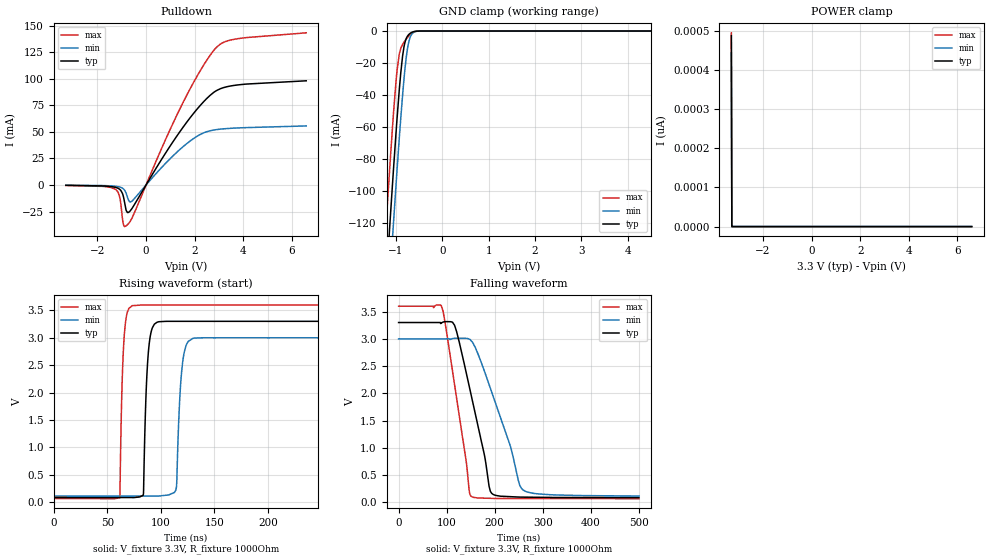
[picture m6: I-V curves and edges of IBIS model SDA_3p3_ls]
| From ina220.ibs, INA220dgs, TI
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|   Model
[Model]   SDA_3p3_ls
Model_type   I/O_open_drain
Polarity   Non-Inverting
Enable   Active-Low
Vinl = 0.99
Vinh = 2.31
Vmeas = 1.65
Vref = 3.3
Cref = 1pF
Rref = 1000
|   typ   min   max
C_comp   2.2433820E-12   1.9359850E-12 2.5433970E-12
[Voltage Range]   3.3   3   3.6
[Temperature Range]   27   85   -40
[Pullup Reference]   3.3   3   3.6
[Pulldown Reference]   -0   -0   -0
[Power Clamp Reference]   3.3   3   3.6
[GND Clamp Reference]   -0   -0   -0
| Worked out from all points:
|   slope of the pulldown table from 0 to 0.495 V, typ, clamps not added: 26.3 ohm
|   GND clamp passes 1 mA (typ) near -0.67 V on its own axis
|   falling waveform, V_fixture 3.3V, R_fixture 1000Ohm: 20-80 % time 47.7ns typ, 63.9ns min, 36.4ns max; typ from 3.3 V to 0.084 V
|   rising waveform, V_fixture 3.3V, R_fixture 1000Ohm: 20-80 % time 3.64ns typ, 4.29ns min, 3.07ns max; typ from 0.083 V to 3.3 V
[Pulldown]
|   Voltage   I(typ)   I(min)   I(max)
-3.3V     -316.9uA   -207.5uA   -421.7uA
-1.261V   -2.207mA   -1.204mA   -4.07mA
-1.102V   -3.787mA   -1.819mA   -9.812mA
-973.5mV  -7.834mA   -2.97mA    -31.07mA
-914.1mV  -12.66mA   -4.043mA   -38.45mA
-825mV    -23.31mA   -7.395mA   -38.56mA
-696.3mV  -25.37mA   -15.33mA   -35.64mA
-587.4mV  -22.38mA   -15.34mA   -31.61mA
1.393V    50.19mA    33.45mA    71.66mA
2.848V    88.14mA    51.95mA    128.4mA
3.61V     93.69mA    53.51mA    137.1mA
6.59V     98.08mA    55.58mA    143.2mA
[GND Clamp]
|   Voltage   I(typ)   I(min)   I(max)
-3.3V     -1.176A    -1.208A    -1.142A
-1.221V   -162.6mA   -196.9mA   -125.6mA
-1.132V   -122mA     -156mA     -85.52mA
-1.073V   -95.72mA   -129.4mA   -60.19mA
-1.053V   -87.15mA   -120.6mA   -52.17mA
-973.5mV  -54.4mA    -86.43mA   -24.47mA
-924mV    -35.97mA   -66.11mA   -14.02mA
-854.7mV  -15.61mA   -39.98mA   -8.368mA
-805.2mV  -7.274mA   -24.13mA   -6.138mA
-755.7mV  -3.503mA   -12.19mA   -4.229mA
-646.8mV  -706.8uA   -1.595mA   -1.161mA
6.59V     0A         0A         0A
[POWER Clamp]
|   Voltage   I(typ)   I(min)   I(max)
-3.3V     487.8pA    443.7pA    495.1pA
-3.28V    0A         0A         0A
-3.27V    0A         0A         0A
6.59V     0A         0A         0A
[Ramp]
R_load = 1000
|   typ   min   max
dV/dt_r   1.93018/3.63153e-09   1.73473/4.27814e-09   2.12159/3.0581e-09
dV/dt_f   1.92984/4.7651e-08   1.73215/6.39826e-08   2.12156/3.64371e-08
[Falling Waveform]
V_fixture = 3.3V
V_fixture_min = 3V
V_fixture_max = 3.6V
R_fixture = 1000Ohm
C_fixture = 0F
|   Time   V(typ)   V(min)   V(max)
0s        3.3V       3V         3.6V
88.8ns    3.289V     3V         3.612V
116.4ns   3.249V     3.01V      2.158V
140.2ns   2.396V     3.009V     774.8mV
146.5ns   2.144V     2.996V     235.6mV
151.5ns   1.946V     2.96V      104.7mV
178.9ns   847mV      2.395V     73.89mV
190.8ns   201.2mV    2.094V     70.74mV
259.4ns   92.79mV    221.6mV    67.74mV
500ns     83.6mV     113.1mV    64.07mV
[Rising Waveform]
V_fixture = 3.3V
V_fixture_min = 3V
V_fixture_max = 3.6V
R_fixture = 1000Ohm
C_fixture = 0F
|   Time   V(typ)   V(min)   V(max)
0s        83.03mV    108.8mV    64.01mV
61.62ns   81.58mV    108.3mV    78.58mV
65.45ns   81.49mV    108.2mV    2.938V
73.15ns   81.3mV     108.2mV    3.585V
83.75ns   155.1mV    108.1mV    3.6V
88.16ns   2.697V     108mV      3.6V
96.49ns   3.284V     108mV      3.6V
114.1ns   3.3V       225.8mV    3.6V
129.9ns   3.3V       2.988V     3.6V
500ns     3.3V       3V         3.6V
